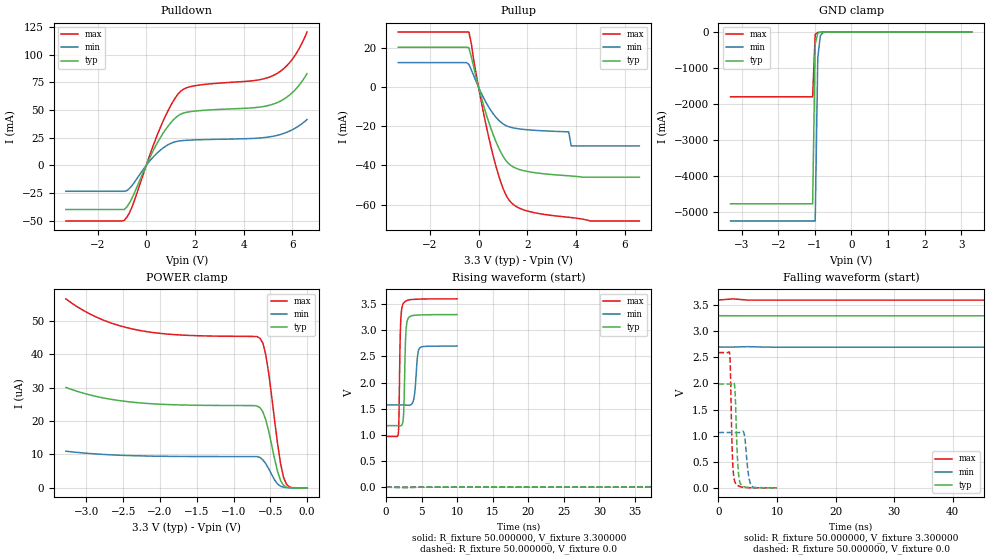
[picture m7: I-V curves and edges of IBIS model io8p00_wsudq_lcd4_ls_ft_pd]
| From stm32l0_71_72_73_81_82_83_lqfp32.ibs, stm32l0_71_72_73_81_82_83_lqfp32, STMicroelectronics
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|   Model io8p00_wsudq_lcd4_ls_ft_pd
[Model]  io8p00_wsudq_lcd4_ls_ft_pd
Model_type I/O
Polarity   Non-Inverting
Enable   Active-Low
Vinl =   0.990000V
Vinh =   2.310000V
Vmeas =  1.650000V
Cref =   50.000000pF
Rref =   100.000000M
Vref =   0.0V
C_comp   3.263700pF   3.224700pF   3.309000pF
[Temperature Range]   25.000000   0.125000k   -40.000000
[Pullup Reference]   3.300000V   2.700000V   3.600000V
[Pulldown Reference]   0.0V   0.0V   0.0V
[POWER Clamp Reference]   3.300000V   2.700000V   3.600000V
[GND Clamp Reference]   0.0V   0.0V   0.0V
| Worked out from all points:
|   slope of the pulldown table from 0 to 0.495 V, typ, clamps not added: 22.6 ohm
|   slope of the pullup table from 0 to 0.495 V, typ, clamps not added: 23.9 ohm
|   GND clamp passes 1 mA (typ) near -0.64 V on its own axis
|   rising waveform, R_fixture 50.000000, V_fixture 3.300000: 20-80 % time 236ps typ, 378ps min, 200ps max; typ from 1.18 V to 3.3 V
|   rising waveform, R_fixture 50.000000, V_fixture 0.0: 20-80 % time 203ns typ, 423ns min, 99.3ns max; typ from 0 V to 1.99 V
|   falling waveform, R_fixture 50.000000, V_fixture 3.300000: 20-80 % time 191ns typ, 382ns min, 105ns max; typ from 3.3 V to 1.18 V
|   falling waveform, R_fixture 50.000000, V_fixture 0.0: 20-80 % time 412ps typ, 576ps min, 337ps max; typ from 1.99 V to 0 V
[Pulldown]
|Voltage   I(typ)   I(min)   I(max)
-3.3V     -39.83mA   -23.37mA   -50.2mA
-900mV    -39.83mA   -23.37mA   -49.53mA
-600mV    -30.28mA   -18.59mA   -38.45mA
500mV     22.11mA    12.28mA    30.1mA
1V        38.33mA    19.81mA    53.88mA
1.4V      46.1mA     22.18mA    66.72mA
2V        49.07mA    23.02mA    71.93mA
4.4V      52.05mA    24.38mA    76.53mA
5.2V      55.25mA    26.3mA     81.02mA
5.6V      59.18mA    28.57mA    86.57mA
6V        65.79mA    32.24mA    95.97mA
6.6V      82.83mA    41.41mA    120.4mA
[Pullup]
|Voltage   I(typ)   I(min)   I(max)
-3.3V     20.5mA     12.63mA    28.27mA
-400mV    20.25mA    11.77mA    28.27mA
-300mV    15.65mA    8.931mA    22.44mA
100mV     -4.685mA   -2.744mA   -6.647mA
600mV     -24.29mA   -13.56mA   -35.12mA
1V        -35.2mA    -18.69mA   -51.62mA
1.4V      -40.6mA    -20.72mA   -59.71mA
2.1V      -43.28mA   -21.83mA   -63.62mA
3.7V      -45.29mA   -22.8mA    -66.5mA
3.8V      -45.39mA   -30mA      -66.64mA
4.6V      -46mA      -30mA      -68.41mA
6.6V      -46mA      -30mA      -68.41mA
[GND_clamp]
|Voltage   I(typ)   I(min)   I(max)
-3.3V     -4.767A    -5.246A    -1.798A
-1.06V    -4.767A    -5.246A    -1.798A
-990mV    -327.3mA   -5.246A    -68.39mA
-920mV    -29.24mA   -722.7mA   -11.25mA
-850mV    -6.784mA   -104.5mA   -6.73mA
-780mV    -3.572mA   -17.39mA   -4.335mA
-500mV    -70.03uA   -187.2uA   -42.37uA
3.28V     73.94uA    88.61uA    51.47uA
[POWER_clamp]
|Voltage   I(typ)   I(min)   I(max)
-3.28V    30.09uA    10.99uA    56.63uA
-2.84V    27.27uA    10.11uA    50.92uA
-2.32V    25.55uA    9.609uA    47.36uA
-640mV    24.06uA    9.1uA      44.84uA
-600mV    22.76uA    8.366uA    43.37uA
-560mV    20.32uA    7.212uA    39.74uA
-520mV    16.86uA    5.676uA    34.15uA
-400mV    4.842uA    1.146uA    13.11uA
-360mV    2.185uA    478.4nA    7.29uA
-320mV    773nA      181.6nA    3.214uA
-240mV    60.58nA    0A         296.5nA
0V        0A         0A         0A
[Ramp]
| variable   typ   min   max
dV/dt_r  1.19400/0.20325u   0.61188/0.42524u   1.55520/99.20259n
dV/dt_f  1.27272/0.19123u   0.63726/0.38190u   1.57835/0.10494u
R_load = 50.000000
[Rising Waveform]
R_fixture= 50.000000
V_fixture= 3.300000
V_fixture_min= 2.700000
V_fixture_max= 3.600000
|time   V(typ)   V(min)   V(max)
0s        1.176V     1.571V     968.8mV
1.702ns   1.176V     1.571V     1.016V
1.802ns   1.174V     1.571V     1.358V
2.022ns   1.172V     1.571V     3.083V
2.382ns   1.276V     1.571V     3.503V
2.743ns   2.866V     1.57V      3.556V
3.063ns   3.218V     1.566V     3.575V
3.884ns   3.283V     1.683V     3.59V
4.725ns   3.292V     2.66V      3.595V
9.97ns    3.299V     2.698V     3.599V
[Rising Waveform]
R_fixture= 50.000000
V_fixture= 0.0
V_fixture_min= 0.0
V_fixture_max= 0.0
|time   V(typ)   V(min)   V(max)
0s        2.466nV    17.32nV    5.594nV
50.05ns   678.8uV    -21.52uV   86.55mV
100.1ns   75.08mV    10.24uV    912.5mV
162.7ns   437mV      5.921mV    1.906V
202.7ns   728.7mV    14.43mV    2.276V
247.7ns   1.042V     47.08mV    2.468V
357.9ns   1.584V     189.3mV    2.573V
503ns     1.879V     441.9mV    2.59V
795.8ns   1.982V     849mV      2.592V
1.246us   1.99V      1.06V      2.592V
[Falling Waveform]
R_fixture= 50.000000
V_fixture= 3.300000
V_fixture_min= 2.700000
V_fixture_max= 3.600000
|time   V(typ)   V(min)   V(max)
0s        3.299V     2.698V     3.599V
82.58ns   3.296V     2.695V     3.488V
150.2ns   3.187V     2.695V     2.484V
212.7ns   2.833V     2.692V     1.574V
250.2ns   2.574V     2.681V     1.217V
285.3ns   2.322V     2.66V      1.082V
390.4ns   1.636V     2.547V     997.7mV
488ns     1.342V     2.387V     979.4mV
838.3ns   1.193V     1.773V     969.4mV
1.246us   1.176V     1.571V     968.8mV
[Falling Waveform]
R_fixture= 50.000000
V_fixture= 0.0
V_fixture_min= 0.0
V_fixture_max= 0.0
|time   V(typ)   V(min)   V(max)
0s        1.99V      1.06V      2.592V
1.922ns   1.99V      1.06V      2.564V
2.402ns   1.996V     1.06V      538.8mV
2.843ns   1.814V     1.06V      106.4mV
3.263ns   528.3mV    1.06V      49.05mV
3.724ns   86.87mV    1.063V     22.83mV
4.404ns   19.04mV    1.026V     7.57mV
5.045ns   7.474mV    313.9mV    4.074mV
5.666ns   3.743mV    35.28mV    2.753mV
9.97ns    2.466nV    17.32nV    5.594nV
